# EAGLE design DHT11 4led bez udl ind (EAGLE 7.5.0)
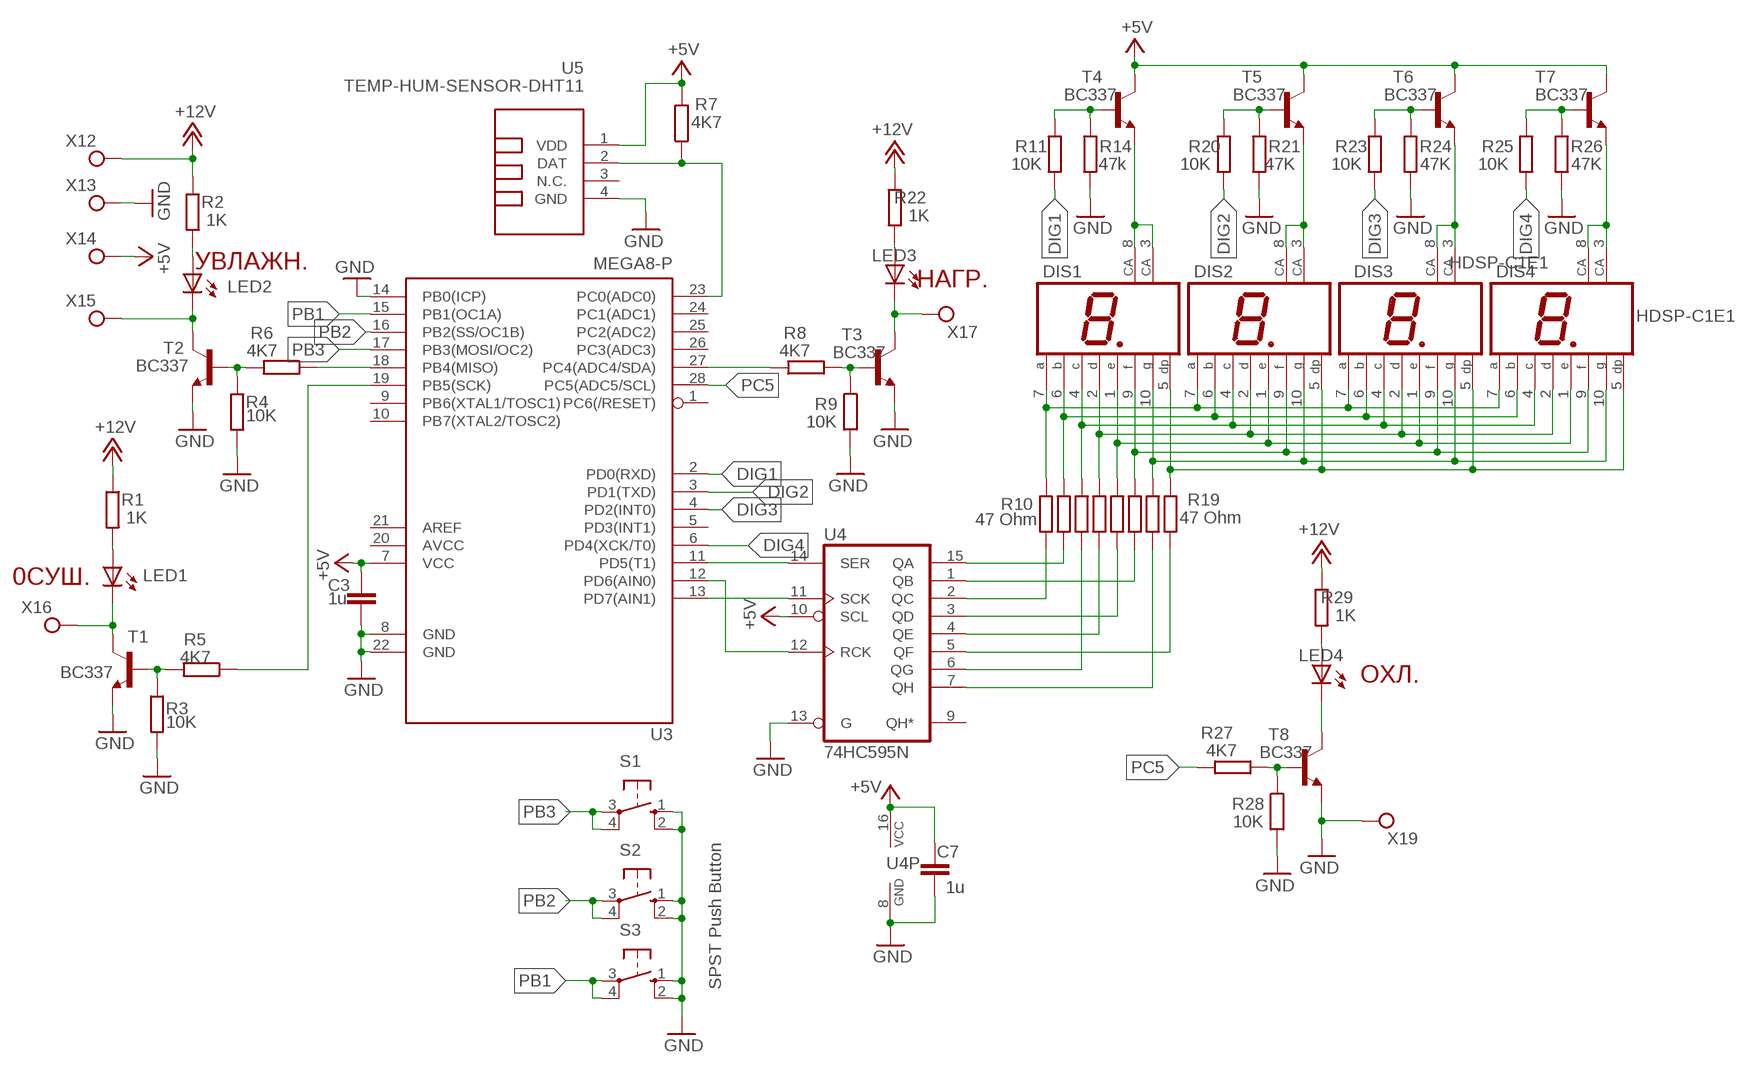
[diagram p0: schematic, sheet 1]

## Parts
C3  1u  C-EUC1206  [C1206]
C7  1u  C-EUC1206  [C1206]
DIS1  HDSP-C1E1  HD-H101  [HDSP-M]
DIS2  HDSP-C1E1  HD-H101  [HDSP-M]
DIS3  HDSP-C1E1  HD-H101  [HDSP-M]
DIS4  HDSP-C1E1  HD-H101  [HDSP-M]
LED1  LED5MM  [LED5MM]
LED2  LED5MM  [LED5MM]
LED3  LED5MM  [LED5MM]
LED4  LED5MM  [LED5MM]
R1  1K  R-EU_0204/7  [0204/7]
R2  1K  R-EU_0204/7  [0204/7]
R3  10K  R-EU_0204/7  [0204/7]
R4  10K  R-EU_0204/7  [0204/7]
R5  4K7  R-EU_0204/7  [0204/7]
R6  4K7  R-EU_0204/7  [0204/7]
R7  4K7  R-EU_0204/7  [0204/7]
R8  4K7  R-EU_0204/7  [0204/7]
R9  10K  R-EU_0204/7  [0204/7]
R10  47 Ohm  R-EU_0204/7  [0204/7]
R11  10K  R-EU_0204/7  [0204/7]
R12  47 Ohm  R-EU_0204/7  [0204/7]
R13  47 Ohm  R-EU_0204/7  [0204/7]
R14  47k  R-EU_0204/7  [0204/7]
R15  47 Ohm  R-EU_0204/7  [0204/7]
R16  47 Ohm  R-EU_0204/7  [0204/7]
R17  47 Ohm  R-EU_0204/7  [0204/7]
R18  47 Ohm  R-EU_0204/7  [0204/7]
R19  47 Ohm  R-EU_0204/7  [0204/7]
R20  10K  R-EU_0204/7  [0204/7]
R21  47K  R-EU_0204/7  [0204/7]
R22  1K  R-EU_0204/7  [0204/7]
R23  10K  R-EU_0204/7  [0204/7]
R24  47K  R-EU_0204/7  [0204/7]
R25  10K  R-EU_0204/7  [0204/7]
R26  47K  R-EU_0204/7  [0204/7]
R27  4K7  R-EU_0204/7  [0204/7]
R28  10K  R-EU_0204/7  [0204/7]
R29  1K  R-EU_0204/7  [0204/7]
S1  SPST Push Button  10-XX  [B3F-10XX]
S2  SPST Push Button  10-XX  [B3F-10XX]
S3  SPST Push Button  10-XX  [B3F-10XX]
T1  BC337  [TO92]
T2  BC337  [TO92]
T3  BC337  [TO92]
T4  BC337  [TO92]
T5  BC337  [TO92]
T6  BC337  [TO92]
T7  BC337  [TO92]
T8  BC337  [TO92]
U3  MEGA8-P  [DIL28-3]
U4  74HC595N  [DIL16]
U5  TEMP-HUM-SENSOR-DHT11  [TEMP-HUM-SENSOR-DHT11]
X12  TPPAD1-17Y  [P1-17Y]
X13  TPPAD1-17Y  [P1-17Y]
X14  TPPAD1-17Y  [P1-17Y]
X15  TPPAD1-17Y  [P1-17Y]
X16  TPPAD1-17Y  [P1-17Y]
X17  TPPAD1-17Y  [P1-17Y]
X19  TPPAD1-17Y  [P1-17Y]

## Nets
+5V: C3.1 C7.1 R7.2 T4.3(C) T5.3(C) T6.3(C) T7.3(C) U3.7(VCC) U4.10(SCL) U4.16(VCC) U5.1(VDD) X14.TP
+12V: R1.1 R2.1 R22.1 R29.1 X12.TP
DIG1: R11.1 U3.2(PD0(RXD))
DIG2: R20.1 U3.3(PD1(TXD))
DIG3: R23.1 U3.4(PD2(INT0))
DIG4: R25.1 U3.6(PD4(XCK/T0))
GND: C3.2 C7.2 R3.2 R4.2 R9.2 R14.1 R21.1 R24.1 R26.1 R28.2 S1.1(S) S1.2(S1) S2.1(S) S2.2(S1) S3.1(S) S3.2(S1) T1.1(E) T2.1(E) T3.1(E) T8.1(E) U3.8(GND) U3.14(PB0(ICP)) U3.22(GND) U4.8(GND) U4.13(G) U5.4(GND) X13.TP X19.TP
N$1: DIS1.7(A) DIS2.7(A) DIS3.7(A) DIS4.7(A) R10.2
N$2: DIS1.6(B) DIS2.6(B) DIS3.6(B) DIS4.6(B) R12.2
N$3: DIS1.4(C) DIS2.4(C) DIS3.4(C) DIS4.4(C) R13.2
N$4: DIS1.2(D) DIS2.2(D) DIS3.2(D) DIS4.2(D) R15.2
N$5: DIS1.1(E) DIS2.1(E) DIS3.1(E) DIS4.1(E) R16.2
N$6: DIS1.9(F) DIS2.9(F) DIS3.9(F) DIS4.9(F) R17.2
N$7: DIS1.10(G) DIS2.10(G) DIS3.10(G) DIS4.10(G) R18.2
N$8: DIS1.5(DP) DIS2.5(DP) DIS3.5(DP) DIS4.5(DP) R19.2
N$9: DIS1.3(CA) DIS1.8(CA) T4.1(E)
N$10: DIS2.3(CA) DIS2.8(CA) T5.1(E)
N$11: R11.2 R14.2 T4.2(B)
N$12: R20.2 R21.2 T5.2(B)
N$13: DIS3.3(CA) DIS3.8(CA) T6.1(E)
N$14: DIS4.3(CA) DIS4.8(CA) T7.1(E)
N$15: R23.2 R24.2 T6.2(B)
N$16: R25.2 R26.2 T7.2(B)
N$17: U3.13(PD7(AIN1)) U4.11(SCK)
N$18: R8.2 R9.1 T3.2(B)
N$19: U3.11(PD5(T1)) U4.14(SER)
N$20: R27.2 R28.1 T8.2(B)
N$21: R5.1 U3.19(PB5(SCK))
N$22: LED1.A R1.2
N$23: LED1.K(C) T1.3(C) X16.TP
N$24: LED2.A R2.2
N$25: U3.12(PD6(AIN0)) U4.12(RCK)
N$26: LED2.K(C) T2.3(C) X15.TP
N$27: R12.1 U4.15(QA)
N$28: LED3.A R22.2
N$29: LED3.K(C) T3.3(C) X17.TP
N$30: LED4.A R29.2
N$31: R17.1 U4.1(QB)
N$32: R10.1 U4.2(QC)
N$33: R16.1 U4.3(QD)
N$34: R15.1 U4.4(QE)
N$35: R19.1 U4.5(QF)
N$36: R13.1 U4.6(QG)
N$37: R18.1 U4.7(QH)
N$38: R8.1 U3.27(PC4(ADC4/SDA))
N$39: LED4.K(C) T8.3(C)
N$40: R4.1 R6.2 T2.2(B)
N$42: R6.1 U3.18(PB4(MISO))
N$47: R3.1 R5.2 T1.2(B)
N$54: R7.1 U3.23(PC0(ADC0)) U5.2(DAT)
PB1: S3.3(P) S3.4(P1) U3.15(PB1(OC1A))
PB2: S2.3(P) S2.4(P1) U3.16(PB2(SS/OC1B))
PB3: S1.3(P) S1.4(P1) U3.17(PB3(MOSI/OC2))
PC5: R27.1 U3.28(PC5(ADC5/SCL))
Unconnected: U3.1(PC6(/RESET)) U3.5(PD3(INT1)) U3.9(PB6(XTAL1/TOSC1)) U3.10(PB7(XTAL2/TOSC2)) U3.21(AREF) U3.24(PC1(ADC1)) U3.25(PC2(ADC2)) U3.26(PC3(ADC3)) U4.9(QH*) U5.3(N.C.)

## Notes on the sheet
- УВЛАЖН.
- НАГР.
- 0СУШ.
- ОХЛ.

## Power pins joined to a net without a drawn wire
AVCC: U3.20(AVCC)

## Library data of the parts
C3 C7 = rcl:C-EU: CAPACITOR, European symbol
DIS1-DIS4 = display-hp:HD-H101: LED DISPLAY Common Anode 7 Segment LED Display, Red, 20 mA, 4 V, 12 mcd, 1, 25.4 m; OC_FARNELL: unknown; OC_NEWARK: unknown
LED1-LED4 = led:LED: LED
R1-R29 = rcl:R-EU_: RESISTOR, European symbol
S1-S3 = switch-omron:10-XX: OMRON SWITCH; MPN: B3F-1000; OC_FARNELL: 176432; OC_NEWARK: 36M3542
T1-T8 = transistor:BC337: NPN TRANSISTOR
U3 = atmel:MEGA8-P: MICROCONTROLLER 8 Kbytes FLASH, 1 kbytes SRAM, 512 bytes EEPROM, USART, 4-channel 10 bit ADC, 2-channel 8 bit ADC Pin compatible with Atmega48, ATMega88, ATMega168 Source: avr.lbr; OC_FARNELL: unknown; OC_NEWARK: unknown
U4 = 74xx-eu:74*595: 8-bit SHIFT REGISTER, output latch
U5 = diy-modules:TEMP-HUM-SENSOR-DHT11: DHT11 - digital humidity & temperature sensor DHT11 datasheet available here: https://akizukidenshi.com/download/ds/aosong/DHT11.pdf Click here to find device on ebay.com
X12-X17 X19 = testpad:TP: Test pad

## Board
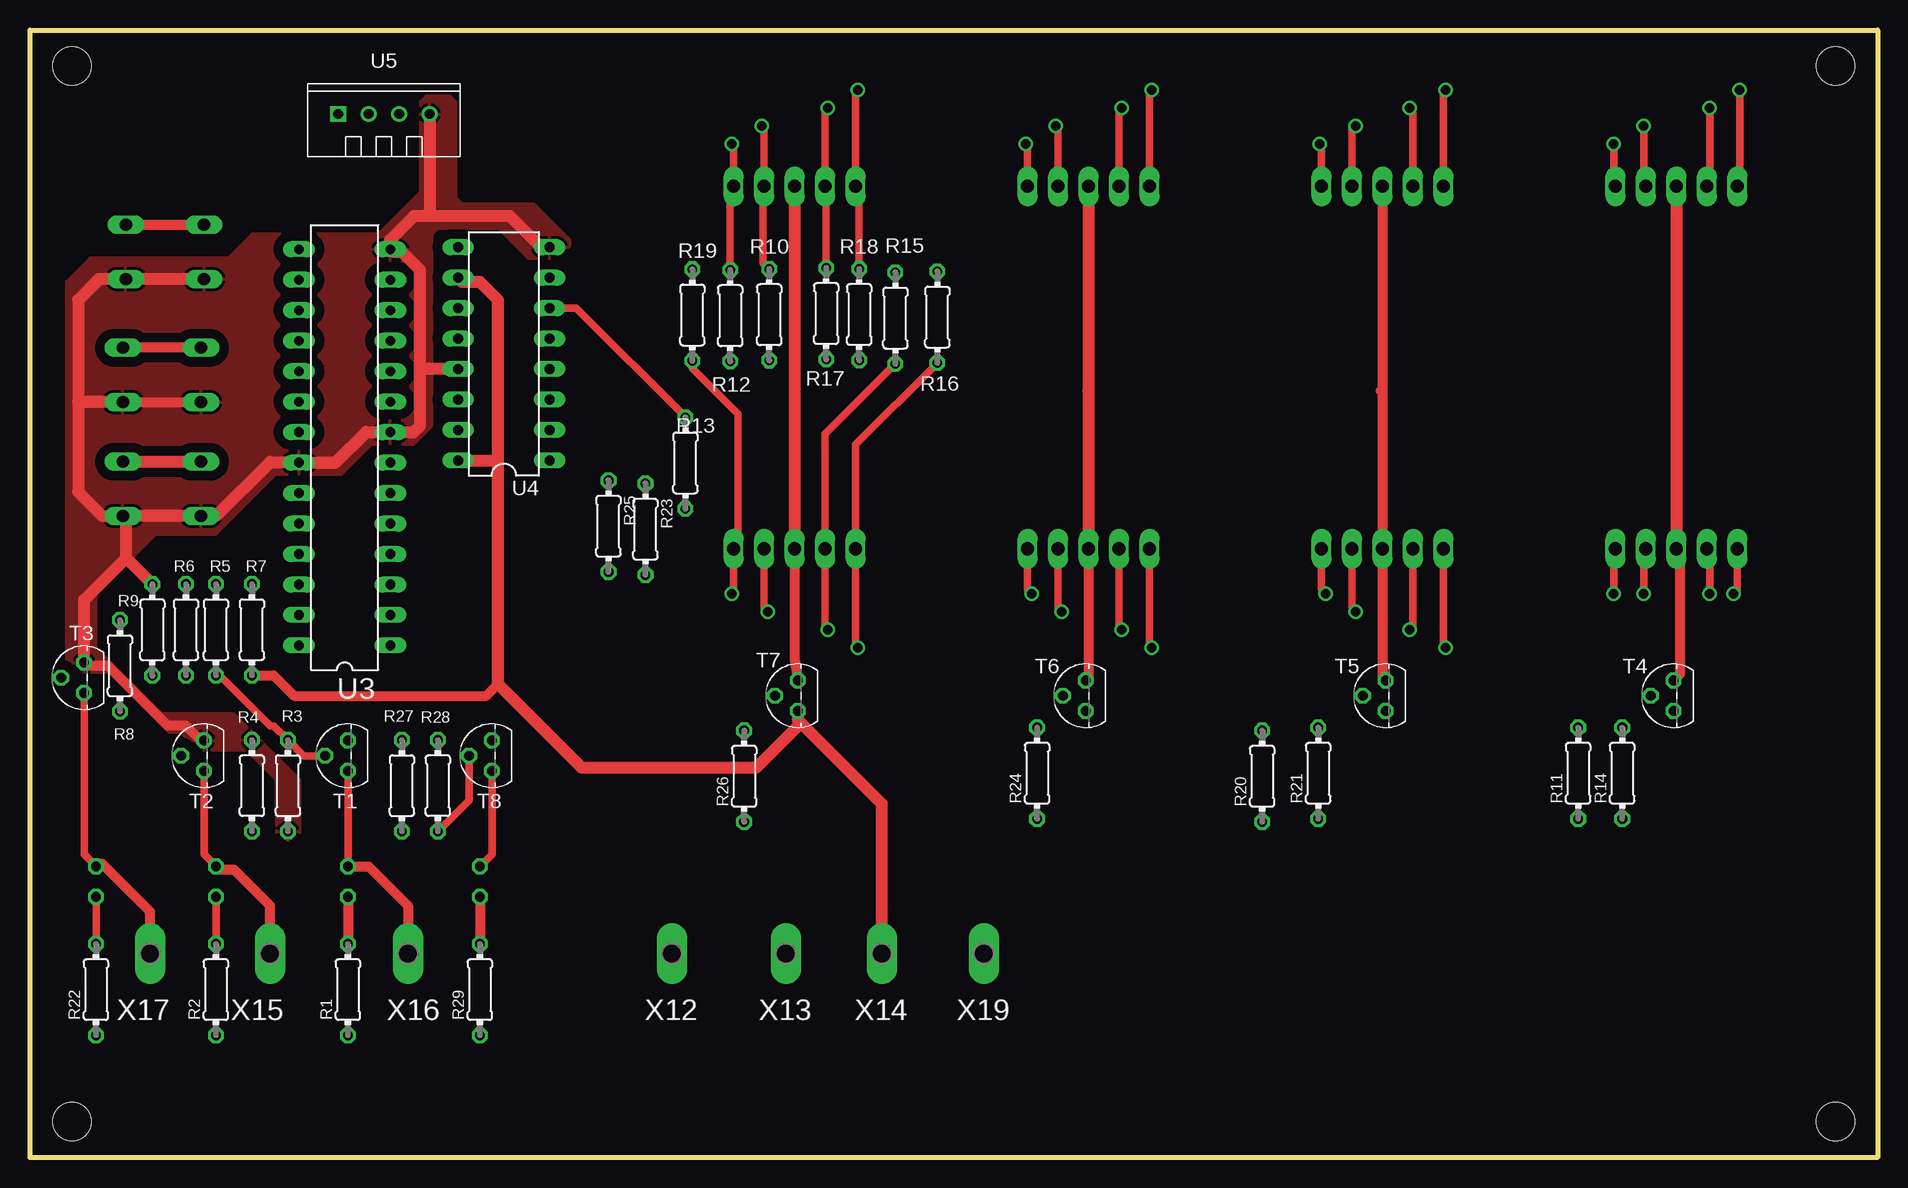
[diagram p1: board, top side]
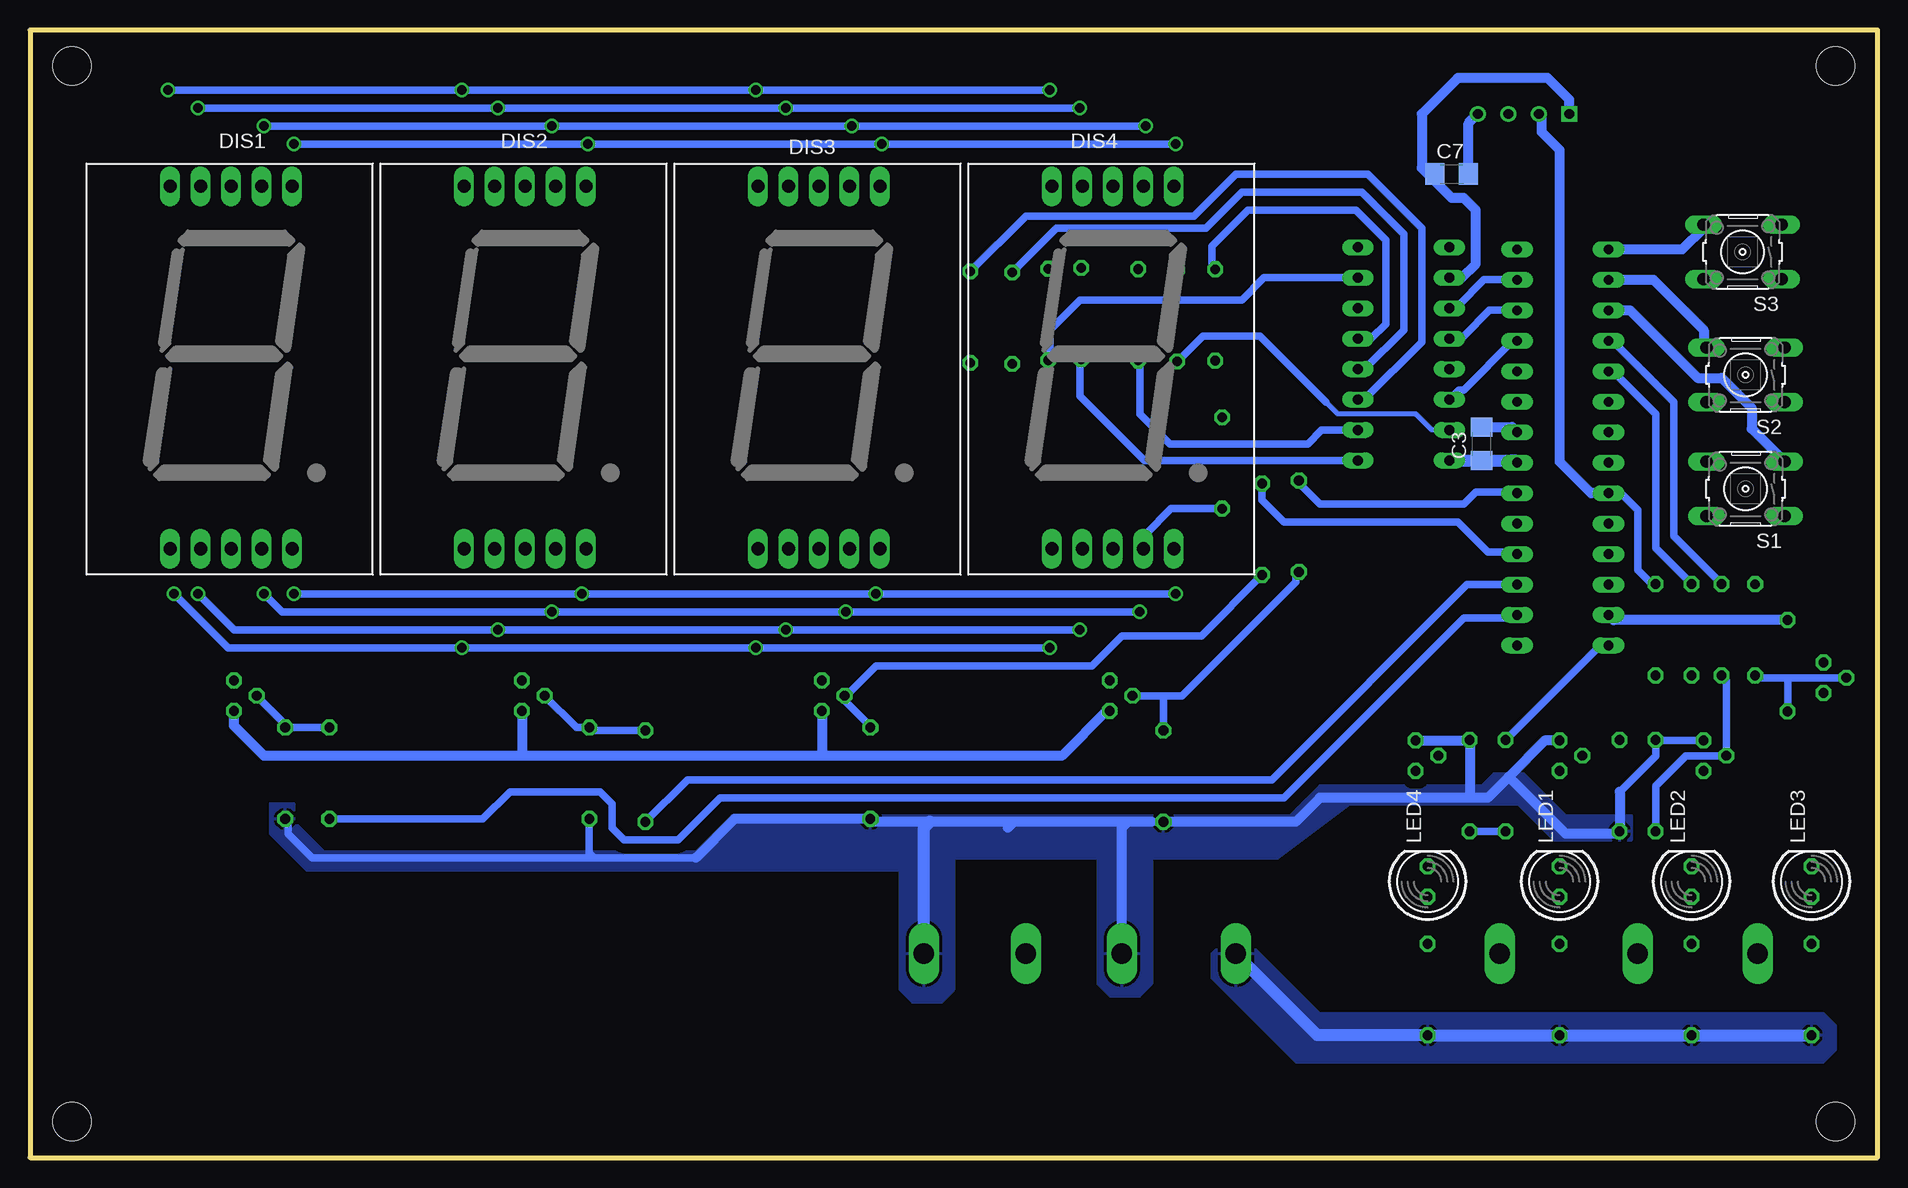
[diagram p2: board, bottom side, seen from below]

Size 154 x 94 mm. Coordinates in mm from the lower left corner, seen from the top.
Outline: 0,0 0,94 154,94 154,0 0,0
Copper layers (1*16): Top 0.035mm / dielectric 1.5mm / Bottom 0.035mm
Design rules "default": minimum track width 10mil, minimum drill 24mil, track to track 8mil, track to pad 8mil, pad to pad 8mil, via to via 8mil, smd to smd 8mil, copper to edge 40mil, drill to drill 8mil, minimum pad ring 10mil, minimum via ring 8mil, stop-mask expansion 4mil, vias tented up to drill 0mil, thermal gap 10mil
Holes 3.2 mm at 3.5,91 150.5,91 3.5,3 150.5,3

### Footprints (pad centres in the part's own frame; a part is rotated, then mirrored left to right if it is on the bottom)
C1206 = smd 1.6 x 1.8: 1 -1.4,0; 2 1.4,0
HDSP-M = drill 1.1 long: 1 -4.318,-16.256; 2 -1.778,-16.256; 3 0.762,-16.256; 4 3.302,-16.256; 5 5.842,-16.256; 6 5.842,13.97; 7 3.302,13.97; 8 0.762,13.97; 9 -1.778,13.97; 10 -4.318,13.97
LED5MM = drill 0.813 octagon: A -1.27,0; K 1.27,0
0204/7 = drill 0.813 octagon: 1 -3.81,0; 2 3.81,0
B3F-10XX = drill 1.016 long: 1 -3.251,2.261; 2 3.251,2.261; 3 -3.251,-2.261; 4 3.251,-2.261
TO92 = drill 0.813 octagon: 1 1.27,0; 2 0,1.905; 3 -1.27,0
DIL28-3 = drill 0.813 long: 1 -16.51,-3.81; 2 -13.97,-3.81; 3 -11.43,-3.81; 4 -8.89,-3.81; 5 -6.35,-3.81; 6 -3.81,-3.81; 7 -1.27,-3.81; 8 1.27,-3.81; 9 3.81,-3.81; 10 6.35,-3.81; 11 8.89,-3.81; 12 11.43,-3.81; 13 13.97,-3.81; 14 16.51,-3.81; 15 16.51,3.81; 16 13.97,3.81; 17 11.43,3.81; 18 8.89,3.81; 19 6.35,3.81; 20 3.81,3.81; 21 1.27,3.81; 22 -1.27,3.81; 23 -3.81,3.81; 24 -6.35,3.81; 25 -8.89,3.81; 26 -11.43,3.81; 27 -13.97,3.81; 28 -16.51,3.81
DIL16 = drill 0.813 long: 1 -8.89,-3.81; 2 -6.35,-3.81; 3 -3.81,-3.81; 4 -1.27,-3.81; 5 1.27,-3.81; 6 3.81,-3.81; 7 6.35,-3.81; 8 8.89,-3.81; 9 8.89,3.81; 10 6.35,3.81; 11 3.81,3.81; 12 1.27,3.81; 13 -1.27,3.81; 14 -3.81,3.81; 15 -6.35,3.81; 16 -8.89,3.81
TEMP-HUM-SENSOR-DHT11 = drill 0.8 square: 1 -3.81,0 | drill 0.8: 2 -1.27,0; 3 1.27,0; 4 3.81,0
P1-17Y = drill 1.702 pad 2.121 long: TP 0,0

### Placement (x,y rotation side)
C3  33,59.5 90 bottom
C7  35.5,82 0 bottom
DIS1  138,67 0 bottom
DIS2  113.5,67 0 bottom
DIS3  89,67 0 bottom
DIS4  64.5,67 0 bottom
LED1  26.5,23 90 bottom
LED2  15.5,23 90 bottom
LED3  5.5,23 90 bottom
LED4  37.5,23 90 bottom
R1  26.5,14 90 top
R2  15.5,14 90 top
R3  21.5,31 270 top
R4  18.5,31 90 top
R5  15.5,44 270 top
R6  13,44 270 top
R7  18.5,44 270 top
R8  7.5,41 270 top
R9  10.2,43.99 90 top
R10  61.62,70.26 90 top
R11  129.05,32.04 90 top
R12  58.37,70.18 90 top
R13  54.63,57.9 270 top
R14  132.72,32.04 90 top
R15  72.13,69.98 270 top
R16  75.63,70.06 270 top
R17  66.37,70.36 90 top
R18  69.12,70.28 90 top
R19  55.21,70.24 270 top
R20  102.71,31.79 90 top
R21  107.38,32.04 90 top
R22  5.5,14 90 top
R23  51.3,52.38 270 top
R24  83.95,32.04 90 top
R25  48.22,52.63 270 top
R26  59.53,31.79 90 top
R27  31,31 270 top
R28  34,31 90 top
R29  37.5,14 90 top
S1  11,55.75 180 bottom
S2  11,65.25 180 bottom
S3  11.25,75.5 180 bottom
T1  26.5,33.5 90 top
T2  14.5,33.5 90 top
T3  4.5,40 90 top
T4  137,38.5 90 top
T5  113,38.5 90 top
T6  88,38.5 90 top
T7  64,38.5 90 top
T8  38.5,33.5 90 top
U3  26.23,59.2 90 top
U4  39.5,67 90 top
U5  29.5,87 0 top
X12  53.5,17 180 top
X13  63,17 180 top
X14  71,17 180 top
X15  20,17 180 top
X16  31.5,17 180 top
X17  10,17 180 top
X19  79.5,17 180 top

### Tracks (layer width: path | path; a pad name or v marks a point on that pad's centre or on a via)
+5V
  Top 0.813: R7.2 20.31,40.19 22,38.5 38,38.5 39,39.5
  Top 1.016: U4.16 38.89,58.11 39,58 | 39,58 39,71.5 37.5,73 36,73 36,73.04 U4.10 | T7.3 64,36.5 | 64,36.5 64,36 60.5,32.5 46,32.5 39,39.5 39,58 | X14.TP 71,29.5 64,36.5
  Bottom 0.61: 64.27,37.23 T7.3
  Bottom 0.813: 64.27,37.23 68,33.5 88,33.5 | 88,33.5 113,33.5 | 113,33.5 134.5,33.5 137,36 T4.3 | T5.3 113,33.5 | T6.3 88,33.5 | U5.1 25.69,88.19 27.5,90 35,90 38,87 38,82.5 37.5,82 C7.1 37,81.9 37,81.5 35.5,80 34.5,80 33.5,79 33.5,74.5 34.65,73.35 U4.10 | C3.1 30.51,58.1 30.5,58.11
  Bottom 1.016: U4.16 30.5,58.11 30.22,58.11 U3.7
+12V
  Bottom 1.016: R22.1 R2.1 R1.1 R29.1 46.69,10.19 X12.TP
  pour Bottom: 4.5,12 46.5,12 52.5,18 54.5,18 55.5,17 55.5,15 48.5,8 4.5,8 3.5,9 3.5,11
DIG1
  Bottom 0.61: R11.1 116.27,28.23 114,30.5 106.5,30.5 105.5,29.5 105.5,27.5 104.5,26.5 100,26.5 96.5,30 49.5,30 34.5,45 30.27,45 U3.2
DIG2
  Bottom 0.61: U3.3 34.23,47.77 50.5,31.5 99.19,31.5 R20.1
DIG3
  Bottom 0.61: R23.1 51.3,54.8 49.5,53 35,53 32.5,50.5 30.23,50.5 U3.4
DIG4
  Bottom 0.61: R25.1 48.22,56.22 46.5,54.5 34.5,54.5 33.5,55.5 30.15,55.5 U3.6
GND
  Top 0.813: S2.1 S2.2 | T2.1 14.23,34.77 13,36 11.5,36 6.5,41 4.77,41 T3.1
  Top 1.016: S3.1 S3.2 5.74,73.24 4,71.5 4,63 | 4,63 4,55.5 6,53.5 7.74,53.5 S1.1 | S2.1 4.01,62.99 4,63 | S1.1 S1.2 15.49,53.49 20,58 22.35,58 U3.22 25.43,57.93 28,60.5 30.01,60.5 U3.8 31.97,60.47 32.5,61 32.5,66 | R9.2 8,50 | 8,50 8,53.24 S1.1 | T3.1 4.5,46.5 8,50 | U4.8 42.61,75.89 40,78.5 33,78.5 | 33,78.5 32,78.5 30,76.5 30,75.75 U3.14 30.25,75.5 31,75.5 32.5,74 32.5,66 | U5.4 33.31,78.81 33,78.5 | U4.13 32.77,65.73 32.5,66
  Bottom 0.61: 98.5,25 107,25 | 107,25 130.5,25 132.5,27 132.5,28.01 R14.1 | R21.1 107.38,25.38 107,25 | T2.1 18.46,34.77 R4.2 18.5,33.5 21.5,30.5 R3.2 | 60.5,28 59.55,28 R26.1
  Bottom 0.813: 98.5,25 95.27,28.23 R24.1 83.72,28 79,28 72,28 | 60.5,28 62.5,28 | 62.5,28 72,28 | 72.5,27.5 72,28 | T1.1 27.73,34.77 30.75,31.75 | 30.75,31.75 32.5,30 34,30 | 34,30 46.5,30 48.5,28 59.51,28 R26.1 | T8.1 34.04,34.77 R28.2 34,30 | 21.5,30.5 21.5,27 26,27 30.75,31.75 | C3.2 30.47,60.9 U3.8 | C7.2 34.1,86.21 U5.4 | X13.TP 63,27.5 62.5,28
  Bottom 1.016: X19.TP 79.5,27.5 79,28
  pour Top (isolate 0.813): 45,76.5 42,79.5 36,79.5 35.5,80 35.5,88 35,88.5 33,88.5 32.5,88 32.5,80.5 29,77 18.5,77 16.5,75 5,75 3,73 3,41.5 4,40.5 6.5,40.5 11.5,35.5 12.5,35.5 14,34 18,34 20.5,31.5 20.5,27 21,26.5 22,26.5 22.5,27 22.5,31.5 17,37 11,37 5.5,42.5 5.5,47 10.5,52 15.5,52 20.5,57 26,57 28.5,59.5 32,59.5 33.5,61 33.5,77 34,77.5 39,77.5 41.5,75 44,75 45,76
  pour Bottom (isolate 0.813): 20.5,28.5 26,28.5 29.5,32 32,32 33,31 46.5,31 49,28.5 95.5,28.5 98.5,25.5 129.5,25.5 132,28 132,29.5 134,29.5 134,27 131,24 81.5,24 81.5,14 80.5,13 78,13 77,14 77,25 65,25 65,14.5 64,13.5 61.5,13.5 60.5,14.5 60.5,25 50,25 44,29.5 30,29.5 27,26.5 20.5,26.5
N$1  (via drill 0.8)
  Top 0.61: v61,86 61.2,85.8 DIS4.7 61.12,80.89 61.12,74.57 R10.2 | v134.5,86 134.5,81.17 DIS1.7 | DIS3.7 85.7,85.8 v85.5,86 | DIS2.7 110.2,85.7 v110.5,86
  Top 0.813: 134.62,80.89 DIS1.7
  Bottom 0.61: v61,86 v85.5,86 v110.5,86 v134.5,86
N$2  (via drill 0.8)
  Top 0.61: v58.5,84.5 58.66,84.34 DIS4.6 58.37,80.68 R12.2 | v132,84.5 132,81.13 DIS1.6 | DIS3.6 83.16,84.34 v83,84.5 | DIS2.6 107.66,84.34 v107.5,84.5
  Bottom 0.61: v58.5,84.5 v83,84.5 v107.5,84.5 v132,84.5
N$3  (via drill 0.8)
  Top 0.61: DIS4.4 61.2,45.8 v61.5,45.5 | DIS1.4 134.5,50.55 v134.5,47 134.37,46.87 | DIS3.4 85.7,45.8 v86,45.5 | DIS2.4 110.2,45.8 v110.5,45.5
  Bottom 0.61: v61.5,45.5 v86,45.5 v110.5,45.5 133,45.5 v134.5,47 | R13.2 58.91,54.09 61,52 61,50.94 DIS4.4
N$4  (via drill 0.8)
  Top 0.61: DIS2.2 115.28,44.28 v115,44 | v66.5,44 66.28,44.22 DIS4.2 66.28,60.32 R15.2 | DIS3.2 90.78,44.22 v91,44 | v140,47 140,50.52 DIS1.2
  Bottom 0.61: v66.5,44 v91,44 v115,44 137,44 v140,47
N$5  (via drill 0.8)
  Top 0.61: DIS2.1 117.82,42.68 v118,42.5 | v69,42.5 68.82,42.68 DIS4.1 68.82,59.44 R16.2 | DIS3.1 93.32,42.68 v93.5,42.5 | DIS1.1 142.32,47.32 v142,47
  Bottom 0.61: v69,42.5 v93.5,42.5 v118,42.5 137.5,42.5 v142,47
N$6  (via drill 0.8)
  Top 0.61: v66.5,87.5 66.28,87.28 DIS4.9 66.37,80.88 R17.2 | v140,87.5 140,81.19 DIS1.9 | DIS3.9 90.78,87.28 v91,87.5 | DIS2.9 115.28,87.22 v115,87.5
  Top 0.813: 139.87,80.88 DIS1.9
  Bottom 0.61: v66.5,87.5 v91,87.5 v115,87.5 v140,87.5
N$7  (via drill 0.8)
  Top 0.61: v69,89 68.82,88.82 DIS4.10 69.12,80.67 R18.2 | v142.5,89 142.5,81.15 DIS1.10 | DIS3.10 93.32,88.82 v93.5,89 | DIS2.10 117.82,88.82 v118,89
  Bottom 0.61: v69,89 v93.5,89 v118,89 v142.5,89
N$8  (via drill 0.8)
  Top 0.61: v58.5,47 58.66,47.16 DIS4.5 59,51.09 59,62 55.21,65.79 R19.2 | v132,47 132,50.59 DIS1.5 | DIS3.5 83.16,47.34 v83.5,47 | DIS2.5 107.66,47.34 v108,47
  Bottom 0.61: v58.5,47 v83.5,47 v108,47 v132,47 | DIS4.5 58.26,50.74
N$9
  Top 0.61: 137.5,50.48 DIS1.3 | 137.14,63.9 137.24,64
  Top 0.813: 137.5,50.48 137.5,40.27 T4.1
  Top 1.016: DIS1.8 137.24,64 DIS1.3
N$10
  Top 0.813: DIS2.8 112.74,63.75 | 112.74,63.75 DIS2.3 112.74,40.03 T5.1 | 112.59,63.9 112.74,63.75
N$11
  Bottom 0.61: R11.2 R14.2 132.72,36.12 T4.2
  Bottom 0.813: 135.04,38.45 T4.2
N$12
  Bottom 0.61: R20.2 107.13,35.6 R21.2 108.44,35.85 T5.2
N$13
  Top 0.61: 88.25,51.24 88.24,51.25
  Top 0.813: 88.14,63.9 88.24,64 | DIS3.3 88.24,40.01 T6.1
  Top 1.016: DIS3.8 88.24,64 88.24,51.25 DIS3.3
N$14
  Top 0.813: DIS4.3 63.74,41.53 T7.1
  Top 1.016: DIS4.8 DIS4.3
N$15
  Bottom 0.61: R23.2 56.37,43.5 63,43.5 65.5,41 83.5,41 86,38.5 T6.2 86,38.41 86,38 83.95,35.95 R24.2
N$16
  Bottom 0.61: T7.2 59.5,38.5 | 59.5,38.5 58,38.5 48.5,48 48.5,48.54 R25.2 | R26.2 59.53,38.47 59.5,38.5
N$17
  Bottom 0.61: U3.13 32.83,73.17 35,71 35.5,71 U4.11
N$18
  Bottom 0.61: T3.2 7.5,40 | 7.5,40 10.02,40 R9.1 | R8.2 7.5,40
N$19
  Bottom 0.61: U3.11 30.41,68.09 34.5,64 34.88,64 U4.14
N$20
  Top 0.61: T8.2 36.59,29.79 R28.1
  Bottom 0.61: R27.2 R28.1
N$21
  Bottom 0.61: U3.19 22.05,65.55 18.5,62 18.5,50.81 R5.1
N$22
  Top 0.813: LED1.A R1.2
N$23
  Top 0.61: T1.3 LED1.K
  Top 0.813: LED1.K 28.23,24.27 31.5,21 X16.TP
N$24
  Top 0.61: LED2.A R2.2
N$25
  Bottom 0.61: U3.12 32.37,70.63 34.5,68.5 35.46,68.5 U4.12
N$26
  Top 0.61: T2.3 14.5,25.27 LED2.K
  Top 0.813: X15.TP 20,21 17,24 15.77,24 LED2.K
N$27
  Bottom 0.406: U4.15 37.15,60.65 38.5,62 45,62 46,63
  Bottom 0.61: 46,63 51.5,68.5 56.24,68.5 R12.1
N$28
  Top 0.61: LED3.A R22.2
N$29
  Top 0.61: T3.3 4.5,25.27 LED3.K
  Top 0.813: X17.TP 10,20.5 6,24.5 5.73,24.5 LED3.K
N$30
  Top 0.813: LED4.A R29.2
N$31
  Bottom 0.61: U4.1 61.11,58.11 66.5,63.5 66.5,66.42 R17.1
N$32
  Bottom 0.61: R10.1 61.5,66.33 61.5,62 59,59.5 47.5,59.5 46.35,60.65 U4.2
N$33
  Bottom 0.61: U4.3 42.81,63.19 38,68 38,77.5 42.5,82 53.5,82 57,78.5 71,78.5 R16.1
N$34
  Bottom 0.61: U4.4 42.77,65.73 39.5,69 39.5,77 43,80.5 53,80.5 56,77.5 68.42,77.5 R15.1
N$35
  Bottom 0.61: U4.5 42.23,68.27 41,69.5 41,76.5 43.5,79 52.5,79 55.5,76 55.5,74.34 R19.1
N$36
  Top 0.61: U4.6 45.53,70.81 R13.1
N$37
  Bottom 0.61: U4.7 51.15,73.35 53,71.5 66.5,71.5 69,69 69,66.59 R18.1
N$38
  Bottom 0.813: R8.1 22,44.81 U3.27
N$39
  Top 0.61: T8.3 38.5,25.27 LED4.K
N$40
  Bottom 0.61: R4.1 18.5,31 16,33.5 T2.2 12.6,39.78 R6.2
N$42
  Bottom 0.61: 21.59,68.09 21.59,67.59 17,63 17,51.81 R6.1
  Bottom 0.813: U3.18 21.59,68.09
N$47
  Top 0.61: R5.2 15.81,40.19 20,36 20.31,36 R3.1 22.81,33.5 T1.2
N$54
  Bottom 0.61: R7.1 18.81,47.81 20,49 20,54 21.5,55.5 22.31,55.5 U3.23
  Bottom 0.813: U3.23 23.89,55.39 26.5,58 26.5,84 28,85.5 28,86.77 U5.2
PB1
  Top 0.813: S3.3 S3.4 14.76,77.76 15,78
  Bottom 0.813: U3.15 16.29,75.71 14.5,77.5 S3.4
PB2
  Top 0.813: S2.4 S2.3
  Bottom 0.813: U3.16 18.67,73.17 14.5,69 14.5,67.76 S2.4
PB3
  Top 1.016: S1.3 S1.4
  Bottom 0.813: U3.17 20.63,70.63 15,65 13,65 10.5,62.5 10.5,60.76 S1.3
PC5
  Bottom 0.61: U3.28 23.12,42.69 R27.1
